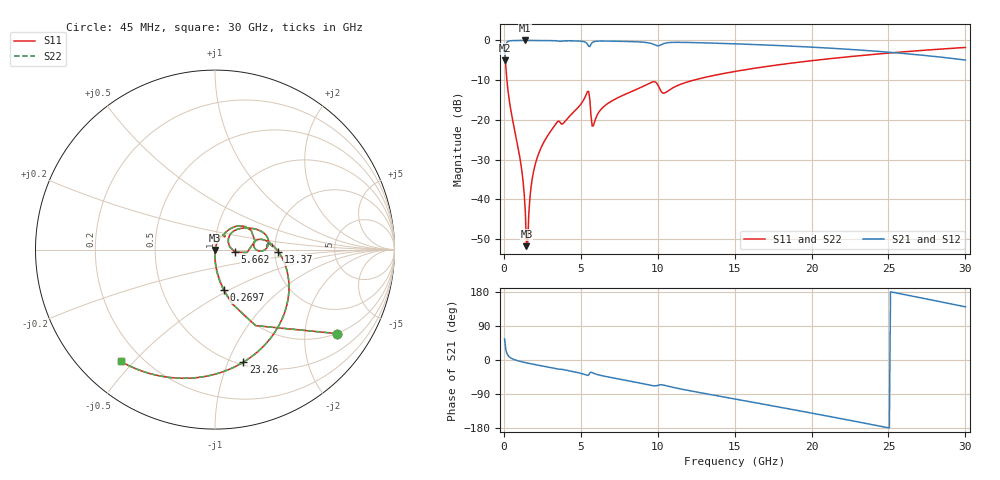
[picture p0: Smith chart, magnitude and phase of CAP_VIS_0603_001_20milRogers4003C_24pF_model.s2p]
! S-parameter model data by Modelithics Inc.  support@modelithics.com  813-866-6335  Tampa FL USA
! S-Parameter data specifications:
! Substrate: 20-mil Rogers 4003C, substrate thickness, H=0.508mm, Dielectric constant, Er=3.75
! PCB Mounting Pad Footprint: Pad width, PadW=0.90mm , Pad length, PadL=1.00mm , Pad gap, PadG (edge-to-edge)=1.00mm , Reference planes=3.0mm apart
! Created Wed Nov 18 13:27:39 2015
# hz S ma R 50
! 2 Port Network Data from SP1.SP block
! freq  magS11  angS11  magS21  angS21  magS12  angS12  magS22  angS22
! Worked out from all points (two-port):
!   401 points, 45 MHz to 30 GHz, reference 50 ohm
!   highest |S21| = -0.01 dB at 1.393 GHz (marker M1); lowest = -5.0 dB at 45 MHz (marker M2)
!   |S21| within 3 dB of the highest: 83.47 MHz to 25.16 GHz (25.07 GHz wide, 199 % of centre)
!   lowest |S11| = -51.7 dB at 1.468 GHz (marker M3), VSWR 1.01, Z = 50.1 - j0.236 ohm
!   |S11| at or under -10 dB: 194.9 MHz to 12.33 GHz (12.14 GHz wide, 194 % of centre)
!   |S22| runs from -51.7 to -1.7 dB; largest |S21 - S12| = 0
!   S11 on the Smith chart (normalised r, x): 45 MHz: 0.99, -2.92; 269.7 MHz: 0.99, -0.47; 5.662 GHz: 1.25, -0.04; 13.37 GHz: 2.09, -0.06; 23.26 GHz: 0.53, -1.14; 30 GHz: 0.12, -0.46
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4.5e7  0.8263 -34.5  0.5631 55.5  0.5631 55.5  0.8263 -34.5
2.696625e8  0.2307 -77.9  0.9724 11.9  0.9724 11.9  0.2307 -77.9
1.093425e9  0.02868 -91.7  0.9983 -4.1  0.9983 -4.1  0.02868 -91.7
1.392975e9  0.006973 -85.9  0.9985 -6.9  0.9985 -6.9  0.006973 -85.9
1.467862e9  0.002587 -65.8  0.9985 -7.6  0.9985 -7.6  0.002587 -65.8
1.617638e9  0.006606 68.6  0.9984 -8.8  0.9984 -8.8  0.006606 68.6
1.917188e9  0.02197 74.6  0.998 -11.3  0.998 -11.3  0.02197 74.6
2.4414e9  0.04586 72.2  0.9969 -15.4  0.9969 -15.4  0.04586 72.2
3.414938e9  0.09148 61.8  0.9875 -23.1  0.9875 -23.1  0.09148 61.8
5.062462e9  0.1639 50.1  0.9747 -35.9  0.9747 -35.9  0.1639 50.1
5.4369e9  0.2281 27.9  0.8936 -40.7  0.8936 -40.7  0.2281 27.9
5.661562e9  0.1133 -7.4  0.8956 -32.3  0.8956 -32.3  0.1133 -7.4
5.886225e9  0.09356 37.4  0.9686 -35.9  0.9686 -35.9  0.09356 37.4
7.2342e9  0.1828 39.9  0.977 -48.3  0.977 -48.3  0.1828 39.9
9.6306e9  0.2991 13.6  0.9086 -67.5  0.9086 -67.5  0.2991 13.6
1.007992e10  0.258 -2.0  0.8591 -66.1  0.8591 -66.1  0.258 -2.0
1.337498e10  0.3535 -2.0  0.9271 -90.8  0.9271 -90.8  0.3535 -2.0
1.50225e10  0.4072 -13.8  0.9056 -103.0  0.9056 -103.0  0.4072 -13.8
2.003996e10  0.5569 -51.0  0.8221 -140.4  0.8221 -140.4  0.5569 -51.0
2.326012e10  0.6464 -75.8  0.7535 -165.2  0.7535 -165.2  0.6464 -75.8
2.505742e10  0.6942 -90.0  0.7095 -179.4  0.7095 -179.4  0.6942 -90.0
3e10  0.815 -130.2  0.5663 140.3  0.5663 140.3  0.815 -130.2
